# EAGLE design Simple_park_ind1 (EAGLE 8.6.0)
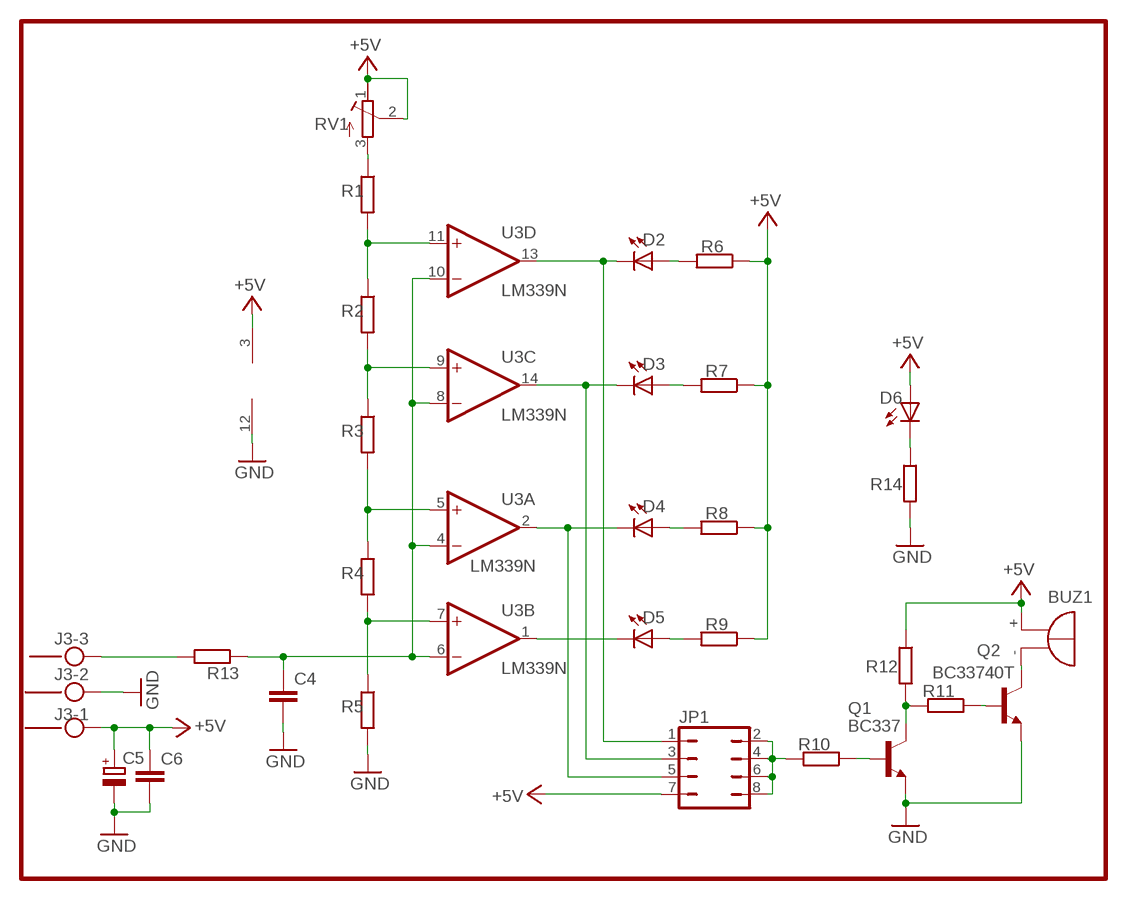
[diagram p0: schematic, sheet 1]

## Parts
BUZ1  F/HMB  [F/HMB]
C4  C-EUC1206  [C1206]
C5  CPOL-EUC/6032-28W  [C/6032-28W]
C6  C-EUC1206  [C1206]
D2  LED5MM  [LED5MM]
D3  LED5MM  [LED5MM]
D4  LED5MM  [LED5MM]
D5  LED5MM  [LED5MM]
D6  LED5MM  [LED5MM]
J3  MKDSN1,5/3-5,08  [MKDSN1,5/3-5,08]
JP1  JP4Q  [JP4Q]
Q1  BC337  [TO92]
Q2  BC33740T  BC337  [TO92]
R1  R-EU_R1206  [R1206]
R2  R-EU_R1206  [R1206]
R3  R-EU_R1206  [R1206]
R4  R-EU_R1206  [R1206]
R5  R-EU_R1206  [R1206]
R6  R-EU_R1206  [R1206]
R7  R-EU_R1206  [R1206]
R8  R-EU_R1206  [R1206]
R9  R-EU_R1206  [R1206]
R10  R-EU_R1206  [R1206]
R11  R-EU_R1206  [R1206]
R12  R-EU_R1206  [R1206]
R13  R-EU_R1206  [R1206]
R14  R-EU_R1206  [R1206]
RV1  R-TRIMM-3386-F  [R-TRIMM-3386F]
U3  LM339N  [DIL14]

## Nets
+5V: BUZ1.+ C5.+ C6.1 D6.A J3.1 JP1.7 R6.1 R7.1 R8.1 R9.1 R12.1 RV1.1(A) RV1.2(S) U3.3(P:V+)
GND: C4.2 C5.- C6.2 J3.2 Q1.1(E) Q2.1(E) R5.2 R14.2 U3.12(P:GND)
N$1: D6.K(C) R14.1
N$2: D5.K(C) U3.1(B:OUT)
N$4: J3.3 R13.2
N$5: C4.1 R13.1 U3.4(A:-IN) U3.6(B:-IN) U3.8(C:-IN) U3.10(D:-IN)
N$6: R1.2 R2.1 U3.11(D:+IN)
N$7: R2.2 R3.1 U3.9(C:+IN)
N$8: R3.2 R4.1 U3.5(A:+IN)
N$9: R4.2 R5.1 U3.7(B:+IN)
N$10: D2.K(C) JP1.1 U3.13(D:OUT)
N$11: D2.A R6.2
N$12: D3.K(C) JP1.3 U3.14(C:OUT)
N$13: D3.A R7.2
N$14: D4.K(C) JP1.5 U3.2(A:OUT)
N$15: D4.A R8.2
N$17: D5.A R9.2
N$18: R1.1 RV1.3(E)
N$19: Q1.2(B) R10.1
N$20: Q1.3(C) R11.2 R12.2
N$21: Q2.2(B) R11.1
N$22: BUZ1.- Q2.3(C)
N$42: JP1.2 JP1.4 JP1.6 JP1.8 R10.2

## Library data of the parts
BUZ1 = buzzer:F/HMB: BUZZER; OC_FARNELL: unknown; OC_NEWARK: unknown
C4 C6 = rcl:C-EU: CAPACITOR, European symbol
C5 = rcl:CPOL-EU: POLARIZED CAPACITOR, European symbol
D2-D6 = led:LED: LED
J3 = con-phoenix-508:MKDSN1,5/3-5,08: MKDSN 1,5/ 3-5,08 Printklemme Nennstrom: 13,5 A Nennspannung: 250 V Rastermaß: 5,08 mm Polzahl: 3 Anschlussart: Schraubanschluss Montage: Löten Anschlussrichtung Leiter/Platine: 0 ° Artikelnummer: 1729131 Source: http://eshop.phoenixcontact.com .. 1729131.pdf
JP1 = jumper:JP4Q: JUMPER
Q1 Q2 = transistor:BC337: NPN TRANSISTOR
R1-R14 = rcl:R-EU_: RESISTOR, European symbol
RV1 = rcl:R-TRIMM-3386-F
U3 = linear:LM339: Low Power Low Offset Voltage Quad Comparators with open collector; LM139/LM239/LM339/LM2901/LM3302

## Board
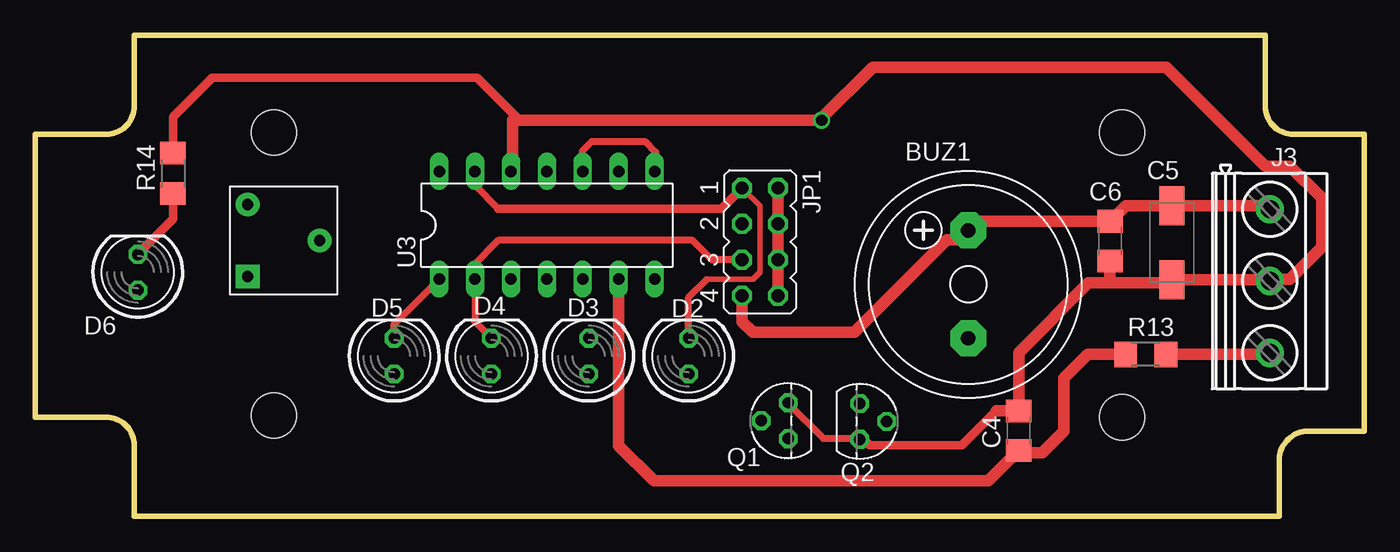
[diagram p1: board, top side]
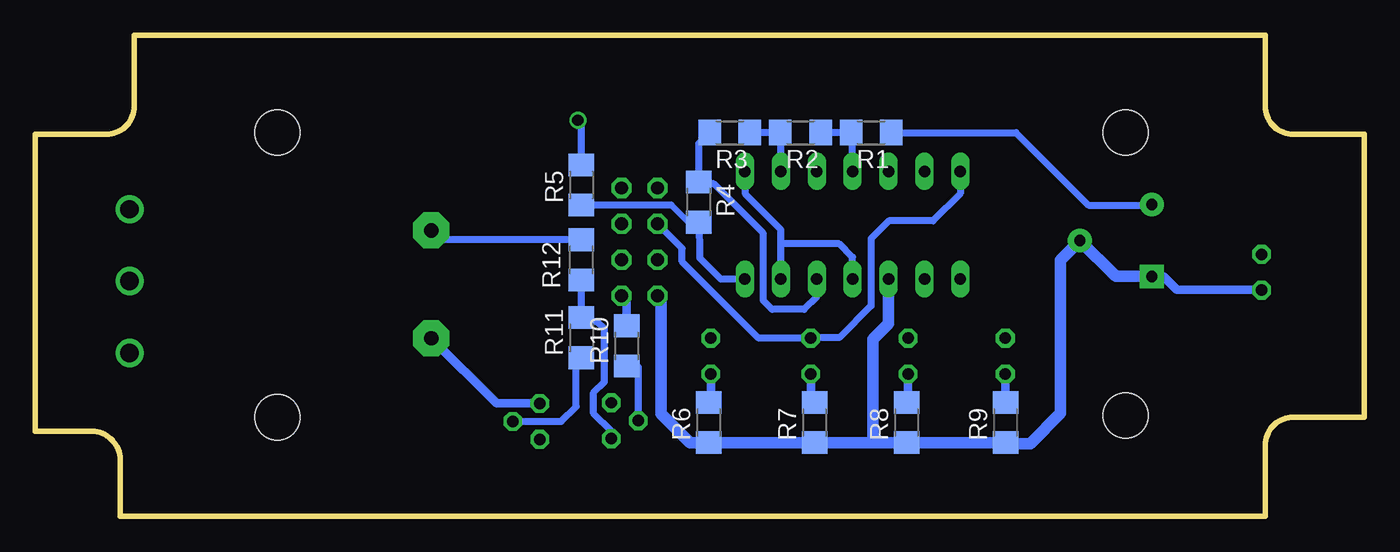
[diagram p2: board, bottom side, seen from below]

Size 94 x 34 mm. Coordinates in mm from the lower left corner, seen from the top.
Outline: 7,0 7,5 arc90 5,7 0,7 0,27 5,27 arc90 7,29 7,34 87,34 87,29 arc90 89,27 94,27 94,6 90,6 arc90 88,4 88,0 7,0
Copper layers (1*16): Top 0.035mm / dielectric 1.5mm / Bottom 0.035mm
Design rules "default": minimum track width 10mil, minimum drill 24mil, track to track 8mil, track to pad 8mil, pad to pad 8mil, via to via 8mil, smd to smd 8mil, copper to edge 40mil, drill to drill 8mil, minimum pad ring 10mil, minimum via ring 8mil, stop-mask expansion 4mil, vias tented up to drill 0mil, thermal gap 10mil
Holes 3.2 mm at 16.88,7.12 76.88,7 16.88,27.12 76.88,27.12

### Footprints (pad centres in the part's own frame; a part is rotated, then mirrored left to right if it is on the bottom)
F/HMB = drill 1.016 pad 2.54 octagon: + 3.81,0; - -3.81,0
C1206 = smd 1.6 x 1.8: 1 -1.4,0; 2 1.4,0
C/6032-28W = smd 2.75 x 1.8: + 2.625,0; - -2.625,0
LED5MM = drill 0.813 octagon: A -1.27,0; K 1.27,0
MKDSN1,5/3-5,08 = drill 1.3 pad 2: 1 -7.641,0.025; 2 -2.561,0.025; 3 2.519,0.025
JP4Q = drill 0.914 octagon: 1 -3.81,-1.27; 2 -3.81,1.27; 3 -1.27,-1.27; 4 -1.27,1.27; 5 1.27,-1.27; 6 1.27,1.27; 7 3.81,-1.27; 8 3.81,1.27
TO92 = drill 0.813 octagon: 1 1.27,0; 2 0,1.905; 3 -1.27,0
R1206 = smd 1.6 x 1.803: 1 -1.422,0; 2 1.422,0
R-TRIMM-3386F = drill 0.8 pad 1.676 square: 1 0,0 | drill 0.8 pad 1.676: 2 5.08,2.54; 3 0,5.08
DIL14 = drill 0.813 long: 1 -7.62,-3.81; 2 -5.08,-3.81; 3 -2.54,-3.81; 4 0,-3.81; 5 2.54,-3.81; 6 5.08,-3.81; 7 7.62,-3.81; 8 7.62,3.81; 9 5.08,3.81; 10 2.54,3.81; 11 0,3.81; 12 -2.54,3.81; 13 -5.08,3.81; 14 -7.62,3.81

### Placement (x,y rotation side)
BUZ1  66,16.39 90 top
C4  69.56,6.04 90 top
C5  80.39,19.34 90 top
C6  76.03,19.45 270 top
D2  46.22,11.31 90 top
D3  39.15,11.31 90 top
D4  32.27,11.31 90 top
D5  25.39,11.31 90 top
D6  7.25,17.25 90 top
J3  87.31,14.06 270 top
JP1  51.26,19.39 270 top
Q1  53.25,6.75 90 top
Q2  58.33,6.71 270 top
R1  34.88,27.12 180 bottom
R2  39.88,27.12 180 bottom
R3  44.88,27.12 180 bottom
R4  47.05,22.2 270 bottom
R5  55.37,23.42 90 bottom
R6  46.38,6.62 90 bottom
R7  38.88,6.62 90 bottom
R8  32.38,6.62 90 bottom
R9  25.38,6.62 90 bottom
R10  52.16,12.04 90 bottom
R11  55.38,12.62 90 bottom
R12  55.38,18.12 270 bottom
R13  78.55,11.45 0 top
R14  9.75,24.25 90 top
RV1  15.03,16.95 0 top
U3  36.19,20.57 0 top

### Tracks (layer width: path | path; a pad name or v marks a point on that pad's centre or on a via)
+5V
  Top 0.813: JP1.7 49.98,13.77 50.75,13 57.95,13 64.5,19.55 65.34,19.55 BUZ1.+ 66.64,20.86 C6.1 77.13,21.96 C5.+ 87.08,21.96 J3.1
  Bottom 0.506: R12.1 65.34,19.55 BUZ1.+
  Bottom 0.61: RV1.1 14.2,16.95 13.25,16 7.27,16 D6.A
  Bottom 0.813: 66.09,20.11 BUZ1.+ | 34.25,5.2 R8.1 R9.1 25.3,5.12 23.62,5.12 21.49,7.26 21.49,18.11 RV1.2 17.57,16.95 RV1.1 | 34.25,5.2 R7.1 R6.1 47.7,5.2 49.75,7.25 49.75,15.35 JP1.7 | U3.3 33.65,13.61 34.75,12.5 34.75,5.7 34.25,5.2
GND  (via drill 0.8)
  Top 0.506: Q1.1 53.25,8 55.75,5.5 58.26,5.5 Q2.1
  Top 0.61: R14.2 9.75,28.25 12.5,31 31.25,31 34.25,28 | Q2.1 58.56,5.43 59,5 65.56,5 68,7.45
  Top 0.813: U3.12 33.75,24.49 33.75,28 34.25,28 v55.62,28 55.62,28.12 59.25,31.75 80,31.75 87,24.75 88.75,24.75 91,22.5 91,19 88.75,16.75 87.45,16.75 J3.2 87.25,16.71 C5.- 80.19,16.5 75.75,16.5 | 68,7.45 C4.2 69.56,11.56 74.5,16.5 75.75,16.5 | C6.2 76.03,16.77 75.75,16.5
  Bottom 0.506: R5.2 55.37,27.74 v55.62,28
N$1
  Top 0.61: R14.1 9.75,21.02 D6.K
N$2
  Top 0.506: D5.K 25.39,13.59 U3.1
N$4
  Top 0.813: R13.2 87.23,11.45 J3.3
N$5
  Top 0.506: U3.10 38.73,25.85 39.38,26.5 43.12,26.5 43.88,25.75 43.88,24.45 U3.8
  Top 0.61: 70.12,4.62 70.25,4.5
  Top 0.813: R13.1 74.44,11.45 72.75,9.75 72.75,6 71.25,4.5 70.25,4.5 69.71,4.5 C4.1 67.42,2.5 43.75,2.5 41.27,4.99 U3.6
  Bottom 0.506: U3.6 41.27,19.38 | 41.27,19.38 41.27,20.27 43.75,22.75 43.75,24.33 U3.8 | U3.4 36.19,18.31 37.12,19.25 41.14,19.25 41.27,19.38
N$6
  Bottom 0.506: R2.1 R1.2 36.19,27.01 U3.11
N$7
  Bottom 0.506: U3.9 41.27,27.09 R2.2 R3.1
N$8
  Bottom 0.506: U3.5 38.73,15.53 39.62,14.62 41.88,14.62 42.5,15.25 42.5,20 46,23.5 46.93,23.5 R4.1 47.05,26.37 R3.2
N$9
  Bottom 0.406: R4.2 47.78,20.78 49,22
  Bottom 0.506: U3.7 45.52,16.77 47,18.25 47,19.23 R4.2 | 49,22 R5.1
N$10
  Top 0.406: 47.5,16.75 50.75,16.75 51.25,17.25 51.25,21.94 JP1.1
  Top 0.506: D2.K 46.22,15.46 47.5,16.75 | U3.13 31.11,23.39 32.75,21.75
  Top 0.61: 32.75,21.75 48.53,21.75 JP1.1
N$11
  Bottom 0.61: D2.A 46.22,8.21 R6.2
N$12
  Bottom 0.506: U3.14 28.57,22.81 30.5,20.88 33.62,20.88 34.88,19.62 34.88,14.88 37.12,12.62 39.1,12.62 D3.K 42.84,12.59 48.25,18 48.25,18.93 JP1.3
N$13
  Bottom 0.61: D3.A 39.15,8.32 R7.2
N$14
  Top 0.506: D4.K 31.11,13.74 U3.2 31,16.87 31,17.75 32.75,19.5 46.5,19.5 47.88,18.12 JP1.5
N$15
  Bottom 0.61: D4.A 32.27,8.16 R8.2
N$17
  Bottom 0.61: D5.A R9.2
N$18
  Bottom 0.506: R1.1 24.62,27.12 19.5,22 15.05,22 RV1.3
N$19
  Bottom 0.506: Q1.2 51.34,10.55 R10.1
N$20
  Bottom 0.506: R12.2 R11.2 55.08,13.75 54.25,13.75 53.75,13.25 53.75,9.5 54.5,8.75 54.5,7.25 53.25,6 Q1.3
N$21
  Bottom 0.506: Q2.2 56.8,6.71 55.75,7.75 55.75,10.83 R11.1
N$22
  Bottom 0.61: Q2.3 61.38,7.97 BUZ1.-
N$42
  Top 0.813: JP1.8 JP1.6 JP1.4 JP1.2
  Bottom 0.61: R10.2 52.16,15.22 JP1.8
